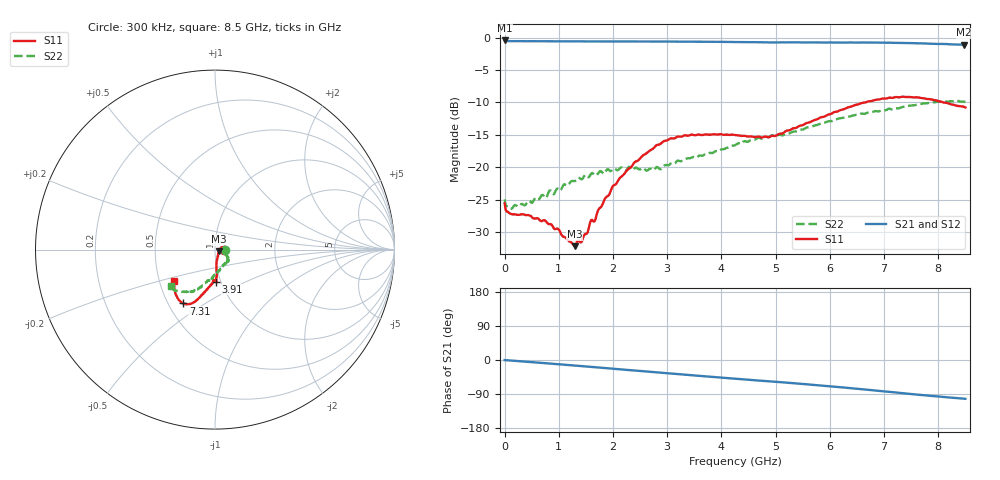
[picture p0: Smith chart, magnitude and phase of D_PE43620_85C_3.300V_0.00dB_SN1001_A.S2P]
! device id: pe43620
! dir: c:\dsa\pe43620\data\pe43620\085c\3p300v\00p00db
! Serial: 1001
! Insertion: A
! Temp: 85C
! VDD: 3.300V
! Attenuation Step: 0.00dB
! IDD: 1.040578e-02mA
! FILE NAME
! DATE 10-22-2008 15:09:12
! CORRECTED  DATA
#  Hz  S  RI  R  50.00
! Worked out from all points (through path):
!   401 points, 300 kHz to 8.5 GHz, reference 50 ohm
!   highest |S21| = -0.44 dB at 300 kHz (marker M1); lowest = -1.1 dB at 8.479 GHz (marker M2)
!   group delay of S21, straight-line fit = 33.2 ps
!   lowest |S11| = -32.2 dB at 1.297 GHz (marker M3), VSWR 1.05, Z = 52.3 - j0.967 ohm
!   |S11| at or under -10 dB: start of sweep to 6.654 GHz; 8.092 GHz to end of sweep
!   |S22| runs from -26.4 to -9.7 dB; largest |S21 - S12| = 0.0052
!   S11 on the Smith chart (normalised r, x): 300 kHz: 1.11, -0.00; 3.91 GHz: 0.95, -0.35; 7.31 GHz: 0.60, -0.41; 8.5 GHz: 0.59, -0.23
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300000  0.0526 -0.0013  0.9508 -0.00378  0.9461 -0.0015  0.0564 -0.00125
1.065463e8  0.0438 0.00199  0.9388 -0.0215  0.9398 -0.0213  0.0479 -0.00426
3.615373e8  0.0421 0.00942  0.9358 -0.0668  0.9366 -0.0673  0.0501 -0.00867
7.440238e8  0.0372 0.0115  0.9273 -0.1365  0.9279 -0.1373  0.055 -0.0189
1.296504e9  0.0228 -0.00923  0.9055 -0.2374  0.9055 -0.2377  0.0678 -0.0389
1.424e9  0.0201 -0.0175  0.8986 -0.2614  0.8987 -0.2611  0.0692 -0.0413
1.593994e9  0.017 -0.0352  0.8882 -0.2914  0.8886 -0.2922  0.0736 -0.0499
1.678991e9  0.0157 -0.0368  0.8829 -0.3071  0.8834 -0.3069  0.0717 -0.0484
2.018979e9  0.00995 -0.0721  0.8586 -0.3687  0.8596 -0.367  0.075 -0.0631
2.401465e9  0.00812 -0.1094  0.8255 -0.4351  0.826 -0.4356  0.0679 -0.0711
2.8477e9  0.0108 -0.149  0.7822 -0.5087  0.7828 -0.5082  0.0464 -0.0861
3.315183e9  0.00325 -0.1759  0.728 -0.5806  0.7284 -0.5805  0.0288 -0.1101
3.910162e9  0.0064 -0.1788  0.6517 -0.6602  0.6516 -0.6606  0.0077 -0.1327
4.25015e9  -0.00133 -0.1771  0.6021 -0.7012  0.6017 -0.7016  -0.00836 -0.1476
4.887628e9  -0.00984 -0.1709  0.5089 -0.7647  0.5071 -0.7656  -0.0292 -0.1689
5.67385e9  -0.0467 -0.2224  0.3811 -0.8336  0.382 -0.8348  -0.0665 -0.1955
6.566318e9  -0.113 -0.2899  0.2104 -0.8921  0.2087 -0.8941  -0.1181 -0.2297
7.09755e9  -0.1581 -0.306  0.0936 -0.9104  0.0913 -0.9101  -0.1511 -0.2398
7.310042e9  -0.1764 -0.3002  0.0467 -0.9096  0.044 -0.9102  -0.1692 -0.2341
8.011267e9  -0.2217 -0.235  -0.0993 -0.8882  -0.1017 -0.8865  -0.2264 -0.228
8.478751e9  -0.2304 -0.1793  -0.1863 -0.8631  -0.1876 -0.8646  -0.2467 -0.2039
8.5e9  -0.2292 -0.1761  -0.1903 -0.8622  -0.1919 -0.8628  -0.2464 -0.2024
